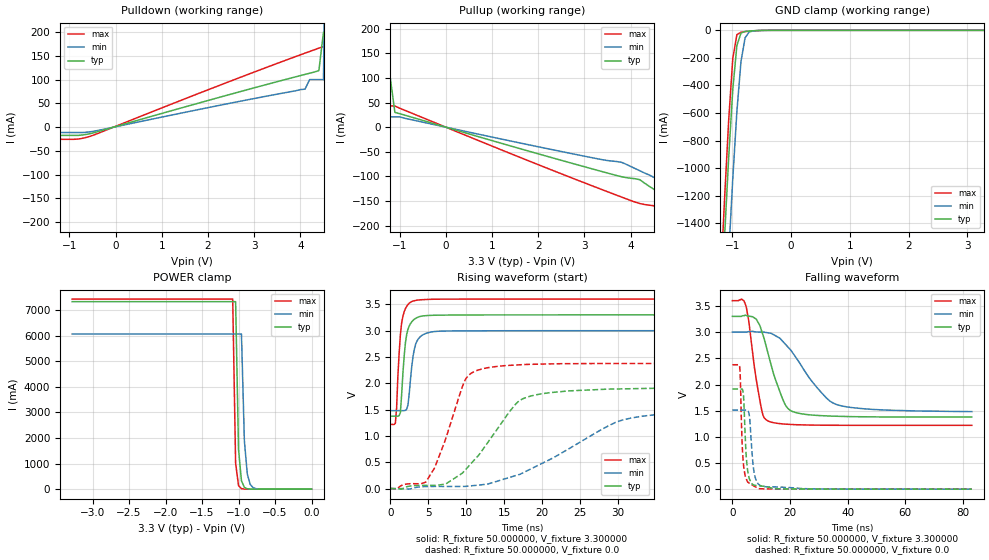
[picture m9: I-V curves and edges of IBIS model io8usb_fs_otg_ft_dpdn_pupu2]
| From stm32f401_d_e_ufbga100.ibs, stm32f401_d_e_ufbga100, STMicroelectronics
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|   Model io8usb_fs_otg_ft_dpdn_pupu2
[Model]  io8usb_fs_otg_ft_dpdn_pupu2
Model_type I/O
Polarity   Non-Inverting
Enable   Active-Low
Vinl =   0.990000V
Vinh =   2.310000V
Vmeas =  1.650000V
Cref =   50.000000pF
Rref =   100.000000M
Vref =   0.0V
C_comp   8.255900pF   7.991100pF   8.650600pF
[Temperature Range]   25.000000   0.125000k   -40.000000
[Pullup Reference]   3.300000V   3.000000V   3.600000V
[Pulldown Reference]   0.0V   0.0V   0.0V
[POWER Clamp Reference]   3.300000V   3.000000V   3.600000V
[GND Clamp Reference]   0.0V   0.0V   0.0V
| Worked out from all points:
|   slope of the pulldown table from 0 to 0.495 V, typ, clamps not added: 36 ohm
|   slope of the pullup table from 0 to 0.495 V, typ, clamps not added: 36.5 ohm
|   GND clamp passes 1 mA (typ) near -0.52 V on its own axis
|   POWER clamp passes 1 mA (typ) near -0.80 V on its own axis
|   rising waveform, R_fixture 50.000000, V_fixture 3.300000: 20-80 % time 665ps typ, 777ps min, 602ps max; typ from 1.38 V to 3.3 V
|   rising waveform, R_fixture 50.000000, V_fixture 0.0: 20-80 % time 6.03ns typ, 11.5ns min, 3.35ns max; typ from 0.005 V to 1.91 V
|   falling waveform, R_fixture 50.000000, V_fixture 3.300000: 20-80 % time 6.38ns typ, 12.3ns min, 3.65ns max; typ from 3.3 V to 1.38 V
|   falling waveform, R_fixture 50.000000, V_fixture 0.0: 20-80 % time 1.15ns typ, 1.41ns min, 972ps max; typ from 1.91 V to 0.005 V
[Pulldown]
|Voltage   I(typ)   I(min)   I(max)
-3.3V     -181mA     -11.29mA   -219mA
-3.2V     -137mA     -11.29mA   -215mA
-2.9V     -124mA     -11.29mA   -198mA
-2.8V     -17.37mA   -11.29mA   -25.6mA
-600mV    -14.67mA   -10.41mA   -20.81mA
4.1V      111mA      80mA       155.7mA
4.2V      113.4mA    100mA      159.2mA
4.4V      119mA      100mA      166.2mA
4.5V      200mA      100mA      169.6mA
4.6V      200mA      1A         173.1mA
4.8V      1A         1A         200mA
6.6V      1A         1A         1A
[Pullup]
|Voltage   I(typ)   I(min)   I(max)
-3.3V     1A         1A         1A
-1.9V     1A         1A         1A
-1.8V     100mA      1A         1A
-1.7V     100mA      1A         100mA
-1.6V     100mA      1A         100mA
-1.5V     100mA      21mA       100mA
-1.3V     100mA      21mA       100mA
-1.2V     100mA      21mA       43mA
-1.1V     30mA       21mA       43mA
4.2V      -106.7mA   -88.5mA    -155mA
5V        -155.8mA   -124mA     -201.9mA
6.6V      -222mA     -161mA     -319mA
[GND_clamp]
|Voltage   I(typ)   I(min)   I(max)
-3.3V     -9.433A    -9.435A    -9.911A
-1.2V     -2.116A    -2.846A    -1.847A
-1.13V    -1.505A    -2.23A     -1.23A
-1.06V    -930.4mA   -1.637A    -658.9mA
-990mV    -432.7mA   -1.08A     -207.3mA
-920mV    -110.5mA   -590.3mA   -31.59mA
-850mV    -19.84mA   -226.8mA   -13.66mA
-780mV    -8.32mA    -54.05mA   -9.516mA
-710mV    -5.29mA    -11.97mA   -6.271mA
-640mV    -3.236mA   -4.296mA   -3.584mA
3.28V     0A         0A         0A
[POWER_clamp]
|Voltage   I(typ)   I(min)   I(max)
-3.28V    7.329A     6.064A     7.431A
-1.08V    7.329A     6.064A     7.431A
-1.04V    7.329A     6.064A     1.016A
-1V       1.545A     6.064A     139.4mA
-960mV    326.1mA    6.064A     19.66mA
-920mV    69.13mA    1.89A      3.273mA
-880mV    14.93mA    589.3mA    1mA
-840mV    3.481mA    183.9mA    655.2uA
-800mV    1.046mA    57.51mA    574.1uA
-720mV    377.9uA    5.818mA    491.6uA
0V        102.7nA    83.74nA    215.4nA
[Ramp]
| variable   typ   min   max
dV/dt_r  1.14565/6.02458n   0.90494/11.43967n   1.42264/3.34658n
dV/dt_f  1.15248/6.37461n   0.90786/12.31529n   1.42698/3.64227n
R_load = 50.000000
[Rising Waveform]
R_fixture= 50.000000
V_fixture= 3.300000
V_fixture_min= 3.000000
V_fixture_max= 3.600000
|time   V(typ)   V(min)   V(max)
0s        1.379V     1.483V     1.221V
667.3ps   1.379V     1.483V     1.242V
834.2ps   1.379V     1.483V     1.534V
1.001ns   1.378V     1.483V     2.135V
1.335ns   1.451V     1.483V     2.926V
1.668ns   2.203V     1.483V     3.276V
2.169ns   2.933V     1.513V     3.464V
3.337ns   3.233V     2.742V     3.573V
7.341ns   3.296V     2.993V     3.598V
83.08ns   3.3V       3V         3.6V
[Rising Waveform]
R_fixture= 50.000000
V_fixture= 0.0
V_fixture_min= 0.0
V_fixture_max= 0.0
|time   V(typ)   V(min)   V(max)
0s        4.597mV    3.98mV     6.081mV
4.671ns   65.14mV    43.2mV     128.1mV
7.174ns   88.36mV    45.48mV    893.9mV
9.843ns   352.5mV    46.38mV    2.058V
12.68ns   844.8mV    86.87mV    2.293V
16.35ns   1.578V     243.8mV    2.347V
17.68ns   1.721V     318.1mV    2.358V
29.7ns    1.894V     1.261V     2.377V
32.87ns   1.902V     1.371V     2.377V
83.08ns   1.914V     1.512V     2.377V
[Falling Waveform]
R_fixture= 50.000000
V_fixture= 3.300000
V_fixture_min= 3.000000
V_fixture_max= 3.600000
|time   V(typ)   V(min)   V(max)
0s        3.3V       3V         3.6V
4.671ns   3.321V     3V         3.507V
9.843ns   3.075V     3V         1.607V
10.84ns   2.906V     2.999V     1.386V
12.35ns   2.6V       2.986V     1.306V
18.02ns   1.651V     2.791V     1.246V
21.69ns   1.47V      2.544V     1.234V
29.36ns   1.411V     1.943V     1.225V
36.37ns   1.394V     1.615V     1.222V
83.08ns   1.379V     1.483V     1.221V
[Falling Waveform]
R_fixture= 50.000000
V_fixture= 0.0
V_fixture_min= 0.0
V_fixture_max= 0.0
|time   V(typ)   V(min)   V(max)
0s        1.914V     1.512V     2.377V
2.503ns   1.914V     1.512V     2.35V
2.669ns   1.914V     1.512V     2.26V
3.504ns   1.906V     1.512V     743.9mV
4.004ns   1.661V     1.512V     401.8mV
4.505ns   954.3mV    1.512V     245.5mV
5.839ns   210.9mV    1.427V     118.5mV
7.341ns   83.2mV     396.5mV    67.95mV
9.009ns   70.71mV    99.81mV    17.22mV
83.08ns   4.597mV    3.98mV     6.081mV
